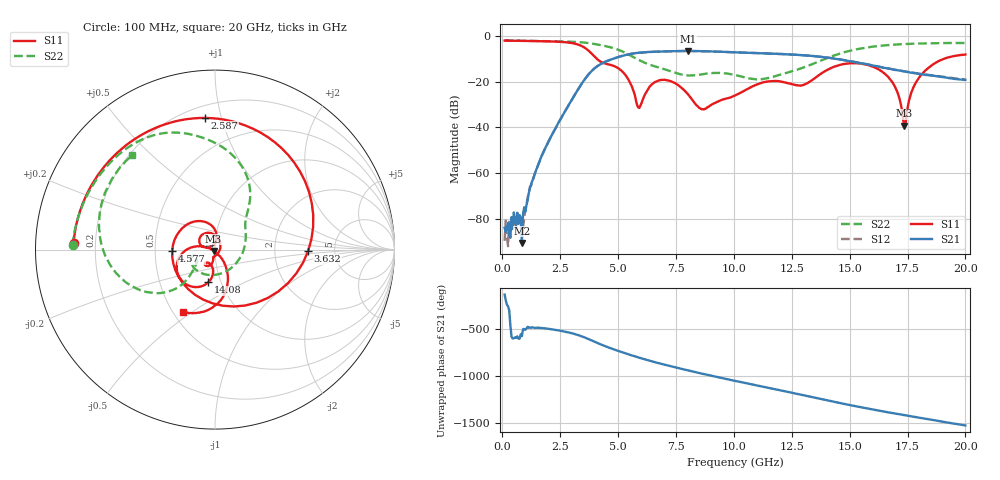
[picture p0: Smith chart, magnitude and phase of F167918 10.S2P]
!  2-Port S-parameters saved by WinCal
! VAR MeasName=S-Parameters (CALIBRATED_DATA) read from VNA (N5242A)
! VAR MeasDate=2016-11-22 10:25:19
! VAR NAME=F167918 10
! VAR FILENAME=F167918 10.S2P
! VAR DATE=2016-11-22 10:25:19
! VAR PHYS_PORTS=1,2
# Hz S DB R 50
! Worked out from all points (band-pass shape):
!   401 points, 100 MHz to 20 GHz, reference 50 ohm
!   highest |S21| = -6.60 dB at 8.01 GHz (marker M1); lowest = -90.6 dB at 846.2 MHz (marker M2)
!   |S21| within 3 dB of the highest: 4.9 GHz to 14.11 GHz (9.212 GHz wide, 96.9 % of centre)
!   lowest |S11| = -39.3 dB at 17.36 GHz (marker M3), VSWR 1.02, Z = 49.2 - j0.755 ohm
!   |S11| at or under -10 dB: 4.078 GHz to 19.08 GHz (15 GHz wide, 130 % of centre)
!   |S22| runs from -19.1 to -2.0 dB; largest |S21 - S12| = 0.004
!   S11 on the Smith chart (normalised r, x): 100 MHz: 0.12, +0.02; 2.587 GHz: 0.28, +0.89; 3.632 GHz: 3.15, -0.07; 4.577 GHz: 0.61, -0.01; 14.08 GHz: 0.87, -0.33; 20 GHz: 0.56, -0.46
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1e8  -2.07 177.3  -83.95 -130.8  -89.65 118.1  -2.00 178.3
8.4625e8  -2.18 157.3  -90.63 145.9  -86.18 -163.1  -2.13 166.5
1.64225e9  -2.32 133.7  -53.89 -125.3  -54.17 -125.3  -2.26 154.0
2.5875e9  -2.67 94.4  -35.12 -159.6  -35.10 -160.1  -2.43 137.3
3.43325e9  -4.46 25.8  -20.85 144.5  -20.88 144.5  -2.81 118.3
3.63225e9  -5.70 -0.9  -18.01 125.2  -18.02 125.3  -3.02 113.1
4.03025e9  -9.53 -71.8  -13.81 82.2  -13.77 82.2  -3.63 102.4
4.5775e9  -12.45 -178.1  -10.80 27.4  -10.77 27.0  -4.75 87.0
5.32375e9  -17.21 98.9  -8.35 -36.2  -8.36 -36.4  -7.47 63.8
5.92075e9  -31.54 131.6  -7.36 -83.2  -7.35 -83.3  -10.66 50.8
6.7665e9  -19.48 144.0  -6.87 -141.4  -6.88 -141.6  -13.89 32.9
8.01025e9  -25.42 61.5  -6.60 143.0  -6.61 142.9  -17.28 -49.8
8.657e9  -32.07 -32.1  -6.69 105.9  -6.70 105.8  -16.78 -103.2
1.005e10  -26.08 -101.4  -7.17 31.1  -7.18 31.2  -17.13 -162.1
1.189075e10  -19.77 -122.4  -7.88 -63.7  -7.87 -63.6  -17.32 -141.7
1.338325e10  -19.35 -96.1  -8.77 -141.7  -8.75 -141.4  -12.38 -133.0
1.407975e10  -14.68 -101.4  -9.54 -178.4  -9.51 -178.4  -9.54 -136.9
1.55225e10  -12.20 -148.2  -12.04 108.9  -11.99 108.7  -5.45 -160.7
1.67165e10  -18.58 171.8  -14.34 54.0  -14.37 54.4  -4.00 177.8
1.736325e10  -39.34 -134.7  -15.58 26.0  -15.50 26.6  -3.57 167.4
1.815925e10  -16.25 -62.8  -16.85 -7.0  -16.71 -6.6  -3.28 155.3
2e10  -8.14 -117.3  -19.24 -83.2  -19.03 -83.6  -3.11 131.3
